| TEXAS INSTRUMENTS INCORPORATED
| Standard Linear and Logic Group
| IBIS Model of sn74CBT16214C
| 12-Bit 1-of-3 FET Multiplexer/demutiplexer with-2V Undershoot- Protection
| This file contains package information for the following:
|  SSOP 56-pin (DL) package as [Component] CBT16214C_DL
|  TSSOP 56-pin (DGG) package as [Component] CBT16214C_DGG
| This device can be powered at the following Vccs:
|  5 volt Vcc
|  4 volt Vcc
| This file provides unique models under the [Model Selector] for each Vcc.
| For operation at a specific Vcc, select the appropriate model after each
| [Model Selector] keyword.
[IBIS Ver]   3.2
[Comment char]  |_char
[File Name]   sn74cbt16214c.ibs
[File Rev]   1.1 | f_die
[Date]   June 9, 2003
[Source]   Data created from TI-SPICE simulations at TI-SLL.
[Notes]   The following is an IBIS list for the CBT16214C.
   Please contact sllibis@ti.com with questions and
   comments concerning SLL IBIS models.
   - Non-monotonic data due to FET characteristics.
   - Power-clamp data has been deleted since there is no
   power-clamp diode in the device.
[Disclaimer] Property of Texas Instruments Incorporated.  Unauthorized
   reproduction and/or distribution is strictly prohibited.
   This product is protected under copyright law.
   Created  2003, (C) Copyright  2003, Texas Instruments
   Incorporated, All Rights Reserved
   UNLESS THERE IS A SIGNED, WRITTEN AGREEMENT TO THE
   CONTRARY, TEXAS INSTRUMENTS (TI) IS PROVIDING THE IBIS
   MODELS  AND WITHOUT ANY WARRANTY, EXPRESSED OR
   IMPLIED.  TI assumes no liability for:
   1) the accuracy of the IBIS models provided to your
   company;
   2) the proper functioning of these IBIS Models in your
   design or for any resulting applications; or
   3) infringement of patents, copyrights or intellectual
   property rights resulting from your use of these IBIS
   models.
   TI provides IBIS Models as a service to our customers.
   You and your company shall not distribute, sell or give
   these models to anyone else without prior written
   permission from TI.
   TI reserves the right to make changes to our products or
   to discontinue any semiconductor product or service
   without notice, and advises our customers to obtain the
   latest version of relevant information to verify, before
   placing orders, that the information being relied on is
   current.
   Please be aware that your receipt and use of the IBIS
   information provided shall serve as acceptance of these
   terms and conditions.  If you do not accept these terms,
   you should return or destroy the IBIS models and any
   other accompanying information immediately.
| Component CBT16214C_DL 56-pin SSOP
[Component]   CBT16214C_DL
[Manufacturer]   Texas Instruments, Inc.
[Package]
|   typ   min   max
R_pkg   5.500e-02   4.800e-02   6.700e-02
L_pkg   6.539e-09   4.803e-09   9.746e-09
C_pkg   8.570e-13   5.000e-13   1.351e-12
[Pin]   signal_name   model_name   R_pin   L_pin   C_pin
1   S0   CBT16214C_IN   6.400e-02   9.646e-09   1.202e-12
2   1A   CBT16214C_IO   5.900e-02   8.723e-09   1.348e-12
3   1B3   CBT16214C_IO   5.900e-02   8.139e-09   1.223e-12
4   2A   CBT16214C_IO   5.600e-02   7.554e-09   1.088e-12
5   2B3   CBT16214C_IO   5.400e-02   6.991e-09   9.660e-13
6   3A   CBT16214C_IO   5.300e-02   6.659e-09   9.730e-13
7   3B3   CBT16214C_IO   5.500e-02   6.321e-09   9.050e-13
8   GND   GND   5.600e-02   5.942e-09   7.130e-13
9   4A   CBT16214C_IO   5.700e-02   5.768e-09   6.780e-13
10   4B3   CBT16214C_IO   5.400e-02   5.459e-09   6.310e-13
11   5A   CBT16214C_IO   5.100e-02   5.224e-09   6.380e-13
12   5B3   CBT16214C_IO   4.800e-02   5.088e-09   6.010e-13
13   6A   CBT16214C_IO   5.000e-02   5.021e-09   5.180e-13
14   6B3   CBT16214C_IO   5.100e-02   4.803e-09   5.000e-13
15   7A   CBT16214C_IO   5.100e-02   4.803e-09   5.000e-13
16   7B3   CBT16214C_IO   5.000e-02   5.021e-09   5.180e-13
17   VCC   POWER   4.800e-02   5.088e-09   6.010e-13
18   8A   CBT16214C_IO   5.100e-02   5.224e-09   6.380e-13
19   GND   GND   5.400e-02   5.459e-09   6.310e-13
20   8B3   CBT16214C_IO   5.700e-02   5.768e-09   6.770e-13
21   9A   CBT16214C_IO   5.500e-02   5.942e-09   7.150e-13
22   9B3   CBT16214C_IO   5.500e-02   6.321e-09   9.070e-13
23   10A   CBT16214C_IO   5.300e-02   6.659e-09   9.720e-13
24   10B3   CBT16214C_IO   5.400e-02   6.991e-09   9.660e-13
25   11A   CBT16214C_IO   5.600e-02   7.554e-09   1.087e-12
26   11B3   CBT16214C_IO   5.900e-02   8.139e-09   1.223e-12
27   12A   CBT16214C_IO   5.900e-02   8.727e-09   1.351e-12
28   12B3   CBT16214C_IO   6.700e-02   9.746e-09   1.210e-12
29   12B2   CBT16214C_IO   6.300e-02   9.630e-09   1.203e-12
30   12B1   CBT16214C_IO   6.000e-02   8.751e-09   1.349e-12
31   11B2   CBT16214C_IO   6.000e-02   8.184e-09   1.224e-12
32   11B1   CBT16214C_IO   5.600e-02   7.543e-09   1.087e-12
33   10B2   CBT16214C_IO   5.400e-02   7.005e-09   9.690e-13
34   10B1   CBT16214C_IO   5.600e-02   6.714e-09   9.750e-13
35   9B2   CBT16214C_IO   5.800e-02   6.384e-09   9.090e-13
36   9B1   CBT16214C_IO   5.700e-02   5.976e-09   7.170e-13
37   8B2   CBT16214C_IO   5.700e-02   5.743e-09   6.770e-13
38   GND   GND   5.400e-02   5.468e-09   6.310e-13
39   8B1   CBT16214C_IO   5.500e-02   5.329e-09   6.440e-13
40   7B2   CBT16214C_IO   5.200e-02   5.189e-09   6.060e-13
41   7B1   CBT16214C_IO   5.200e-02   5.053e-09   5.190e-13
42   6B2   CBT16214C_IO   5.200e-02   4.825e-09   5.020e-13
43   6B1   CBT16214C_IO   5.400e-02   4.897e-09   5.060e-13
44   5B2   CBT16214C_IO   5.200e-02   5.093e-09   5.210e-13
45   5B1   CBT16214C_IO   5.100e-02   5.179e-09   6.080e-13
46   4B2   CBT16214C_IO   5.400e-02   5.314e-09   6.450e-13
47   4B1   CBT16214C_IO   5.500e-02   5.511e-09   6.320e-13
48   3B2   CBT16214C_IO   5.700e-02   5.770e-09   6.770e-13
49   GND   GND   5.600e-02   5.956e-09   7.160e-13
50   3B1   CBT16214C_IO   5.500e-02   6.320e-09   9.050e-13
51   2B2   CBT16214C_IO   5.200e-02   6.621e-09   9.680e-13
52   2B1   CBT16214C_IO   5.300e-02   6.974e-09   9.660e-13
53   1B2   CBT16214C_IO   5.700e-02   7.571e-09   1.089e-12
54   1B1   CBT16214C_IO   5.700e-02   8.097e-09   1.219e-12
55   S2   CBT16214C_IN   5.900e-02   8.723e-09   1.349e-12
56   S1   CBT16214C_IN   6.100e-02   9.560e-09   1.199e-12
| Component CBT16214C_DGG 56-pin TSSOP
[Component]   CBT16214C_DGG
[Manufacturer]   Texas Instruments, Inc.
[Package]
|   typ   min   max
R_pkg   4.500e-02   3.500e-02   6.200e-02
L_pkg   3.324e-09   2.403e-09   5.094e-09
C_pkg   5.640e-13   3.410e-13   9.140e-13
[Pin]   signal_name   model_name   R_pin   L_pin   C_pin
1   S0   CBT16214C_IN   6.200e-02   5.094e-09   8.560e-13
2   1A   CBT16214C_IO   6.100e-02   4.621e-09   9.020e-13
3   1B3   CBT16214C_IO   6.000e-02   4.316e-09   8.020e-13
4   2A   CBT16214C_IO   5.900e-02   3.968e-09   6.980e-13
5   2B3   CBT16214C_IO   5.700e-02   3.716e-09   6.490e-13
6   3A   CBT16214C_IO   4.200e-02   3.517e-09   6.530e-13
7   3B3   CBT16214C_IO   4.100e-02   3.160e-09   5.700e-13
8   GND   GND   3.900e-02   2.981e-09   4.820e-13
9   4A   CBT16214C_IO   3.900e-02   2.808e-09   4.470e-13
10   4B3   CBT16214C_IO   3.800e-02   2.715e-09   4.090e-13
11   5A   CBT16214C_IO   4.100e-02   2.675e-09   3.910e-13
12   5B3   CBT16214C_IO   3.900e-02   2.536e-09   3.660e-13
13   6A   CBT16214C_IO   3.900e-02   2.457e-09   3.480e-13
14   6B3   CBT16214C_IO   3.800e-02   2.411e-09   3.530e-13
15   7A   CBT16214C_IO   3.900e-02   2.456e-09   3.550e-13
16   7B3   CBT16214C_IO   3.900e-02   2.471e-09   3.490e-13
17   VCC   POWER   4.000e-02   2.580e-09   3.700e-13
18   8A   CBT16214C_IO   3.800e-02   2.651e-09   3.890e-13
19   GND   GND   3.800e-02   2.739e-09   4.110e-13
20   8B3   CBT16214C_IO   3.900e-02   2.838e-09   4.490e-13
21   9A   CBT16214C_IO   3.800e-02   2.988e-09   4.840e-13
22   9B3   CBT16214C_IO   3.800e-02   3.104e-09   5.640e-13
23   10A   CBT16214C_IO   4.000e-02   3.427e-09   6.380e-13
24   10B3   CBT16214C_IO   5.600e-02   3.654e-09   6.410e-13
25   11A   CBT16214C_IO   5.700e-02   3.932e-09   7.000e-13
26   11B3   CBT16214C_IO   5.800e-02   4.257e-09   8.060e-13
27   12A   CBT16214C_IO   5.700e-02   4.580e-09   9.140e-13
28   12B3   CBT16214C_IO   5.900e-02   5.038e-09   8.610e-13
29   12B2   CBT16214C_IO   6.000e-02   5.058e-09   8.580e-13
30   12B1   CBT16214C_IO   5.600e-02   4.543e-09   9.040e-13
31   11B2   CBT16214C_IO   5.700e-02   4.241e-09   8.020e-13
32   11B1   CBT16214C_IO   5.900e-02   3.933e-09   6.990e-13
33   10B2   CBT16214C_IO   5.600e-02   3.616e-09   6.370e-13
34   10B1   CBT16214C_IO   3.700e-02   3.368e-09   6.400e-13
35   9B2   CBT16214C_IO   3.600e-02   3.024e-09   5.630e-13
36   9B1   CBT16214C_IO   3.500e-02   2.876e-09   4.740e-13
37   8B2   CBT16214C_IO   3.500e-02   2.745e-09   4.440e-13
38   GND   GND   3.700e-02   2.683e-09   4.050e-13
39   8B1   CBT16214C_IO   3.800e-02   2.603e-09   3.820e-13
40   7B2   CBT16214C_IO   3.800e-02   2.510e-09   3.620e-13
41   7B1   CBT16214C_IO   3.600e-02   2.412e-09   3.410e-13
42   6B2   CBT16214C_IO   3.800e-02   2.416e-09   3.490e-13
43   6B1   CBT16214C_IO   3.800e-02   2.403e-09   3.490e-13
44   5B2   CBT16214C_IO   3.700e-02   2.429e-09   3.410e-13
45   5B1   CBT16214C_IO   3.600e-02   2.483e-09   3.580e-13
46   4B2   CBT16214C_IO   3.700e-02   2.614e-09   3.810e-13
47   4B1   CBT16214C_IO   3.500e-02   2.669e-09   4.020e-13
48   3B2   CBT16214C_IO   3.600e-02   2.763e-09   4.420e-13
49   GND   GND   3.600e-02   2.942e-09   4.780e-13
50   3B1   CBT16214C_IO   3.500e-02   3.053e-09   5.640e-13
51   2B2   CBT16214C_IO   3.600e-02   3.408e-09   6.410e-13
52   2B1   CBT16214C_IO   5.800e-02   3.698e-09   6.410e-13
53   1B2   CBT16214C_IO   5.900e-02   3.974e-09   6.970e-13
54   1B1   CBT16214C_IO   6.100e-02   4.327e-09   8.020e-13
55   S2   CBT16214C_IN   6.100e-02   4.624e-09   9.050e-13
56   S1   CBT16214C_IN   6.000e-02   5.063e-09   8.580e-13
[Series Switch Groups]
| Function Group States
On  1 /   | 1A->1B1 S0 HIGH S1 LOW S2 LOW
On  2 /   | 1A->1B2 S0 LOW S1 HIGH S2 LOW
On  3 /   | 1A->1B3 S0 HIGH S1 LOW S2 HIGH
Off 1 2 3 /   | DISABLE ALL S0 LOW S1 LOW S2 LOW
[Series Pin Mapping]   pin_2   model_name   function_table_group
2   54   CBT16214C_IO_50_S   1
| 2   54   CBT16214C_IO_40_S   1
4   52   CBT16214C_IO_50_S   1
| 4   52   CBT16214C_IO_40_S   1
6   50   CBT16214C_IO_50_S   1
| 6   50   CBT16214C_IO_40_S   1
9   47   CBT16214C_IO_50_S   1
| 9   47   CBT16214C_IO_40_S   1
11   45   CBT16214C_IO_50_S   1
| 11   45   CBT16214C_IO_40_S   1
13   43   CBT16214C_IO_50_S   1
| 13   43   CBT16214C_IO_40_S   1
15   41   CBT16214C_IO_50_S   1
| 15   41   CBT16214C_IO_40_S   1
18   39   CBT16214C_IO_50_S   1
| 18   39   CBT16214C_IO_40_S   1
21   36   CBT16214C_IO_50_S   1
| 21   36   CBT16214C_IO_40_S   1
23   34   CBT16214C_IO_50_S   1
| 23   34   CBT16214C_IO_40_S   1
25   32   CBT16214C_IO_50_S   1
| 25   32   CBT16214C_IO_40_S   1
27   30   CBT16214C_IO_50_S   1
| 27   30   CBT16214C_IO_40_S   1
2   53   CBT16214C_IO_50_S   2
| 2   53   CBT16214C_IO_40_S   2
4   51   CBT16214C_IO_50_S   2
| 4   51   CBT16214C_IO_40_S   2
6   48   CBT16214C_IO_50_S   2
| 6   48   CBT16214C_IO_40_S   2
9   46   CBT16214C_IO_50_S   2
| 9   46   CBT16214C_IO_40_S   2
11   44   CBT16214C_IO_50_S   2
| 11   44   CBT16214C_IO_40_S   2
13   42   CBT16214C_IO_50_S   2
| 13   42   CBT16214C_IO_40_S   2
15   40   CBT16214C_IO_50_S   2
| 15   40   CBT16214C_IO_40_S   2
18   37   CBT16214C_IO_50_S   2
| 18   37   CBT16214C_IO_40_S   2
21   35   CBT16214C_IO_50_S   2
| 21   35   CBT16214C_IO_40_S   2
23   33   CBT16214C_IO_50_S   2
| 23   33   CBT16214C_IO_40_S   2
25   31   CBT16214C_IO_50_S   2
| 25   31   CBT16214C_IO_40_S   2
27   29   CBT16214C_IO_50_S   2
| 27   29   CBT16214C_IO_40_S   2
2   3   CBT16214C_IO_50_S   3
| 2   3   CBT16214C_IO_40_S   3
4   5   CBT16214C_IO_50_S   3
| 4   5   CBT16214C_IO_40_S   3
6   7   CBT16214C_IO_50_S   3
| 6   7   CBT16214C_IO_40_S   3
9   10   CBT16214C_IO_50_S   3
| 9   10   CBT16214C_IO_40_S   3
11   12   CBT16214C_IO_50_S   3
| 11   12   CBT16214C_IO_40_S   3
13   14   CBT16214C_IO_50_S   3
| 13   14   CBT16214C_IO_40_S   3
15   16   CBT16214C_IO_50_S   3
| 15   16   CBT16214C_IO_40_S   3
18   20   CBT16214C_IO_50_S   3
| 18   20   CBT16214C_IO_40_S   3
21   22   CBT16214C_IO_50_S   3
| 21   22   CBT16214C_IO_40_S   3
23   24   CBT16214C_IO_50_S   3
| 23   24   CBT16214C_IO_40_S   3
25   26   CBT16214C_IO_50_S   3
| 25   26   CBT16214C_IO_40_S   3
27   28   CBT16214C_IO_50_S   3
| 27   28   CBT16214C_IO_40_S   3
| Model CBT16214C_IN
[Model Selector]   CBT16214C_IN
CBT16214C_IN_50   5 volt Vcc
CBT16214C_IN_40   4 volt Vcc
| Model CBT16214C_IO
[Model Selector]   CBT16214C_IO
CBT16214C_IO_50   5 volt Vcc
CBT16214C_IO_40   4 volt Vcc
| Model CBT16214C_IO_S
[Model Selector]   CBT16214C_IO_S
CBT16214C_IO_50_S   5 volt Vcc
CBT16214C_IO_40_S   4 volt Vcc
[Model]   CBT16214C_IO_50_S
Model_type  Series_switch
| variable   typ   min   max
C_comp   0   0   0
[Temperature Range]   40   100   -40
| Ambient temperature   25   85   -40
[Voltage range]   5   4.5   5.5
[On]
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[Off]
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[Model]   CBT16214C_IO_40_S
Model_type  Series_switch
| variable   typ   min   max
C_comp   0   0   0
[Temperature Range]   40   100   -40
| Ambient temperature   25   85   -40
[Voltage range]   4   4   4
[On]
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[Off]
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| Models and submodels in the file (6): CBT16214C_IN_50 (Input), CBT16214C_IN_40 (Input), CBT16214C_IO_50_S (Series_switch), CBT16214C_IO_50 (Terminator), CBT16214C_IO_40_S (Series_switch), CBT16214C_IO_40 (Terminator)
